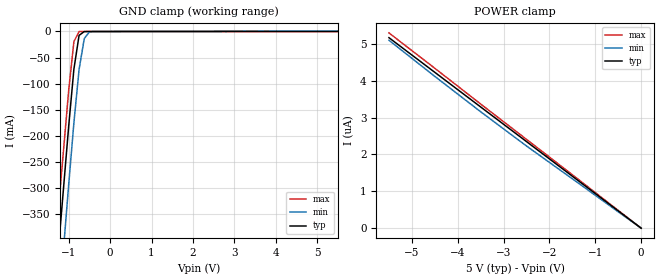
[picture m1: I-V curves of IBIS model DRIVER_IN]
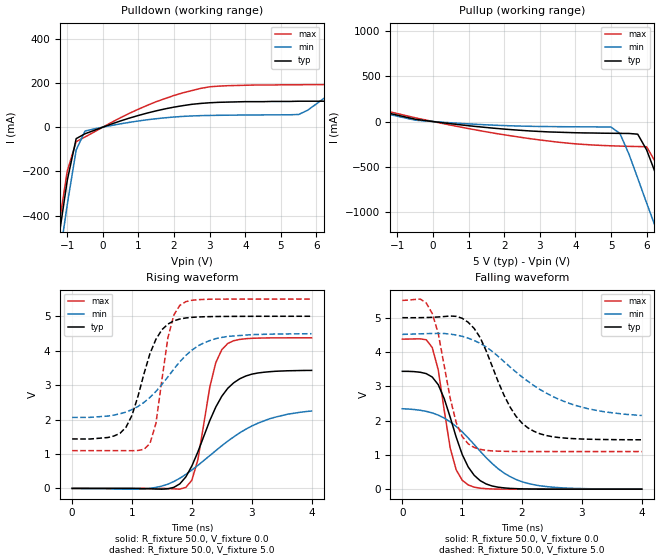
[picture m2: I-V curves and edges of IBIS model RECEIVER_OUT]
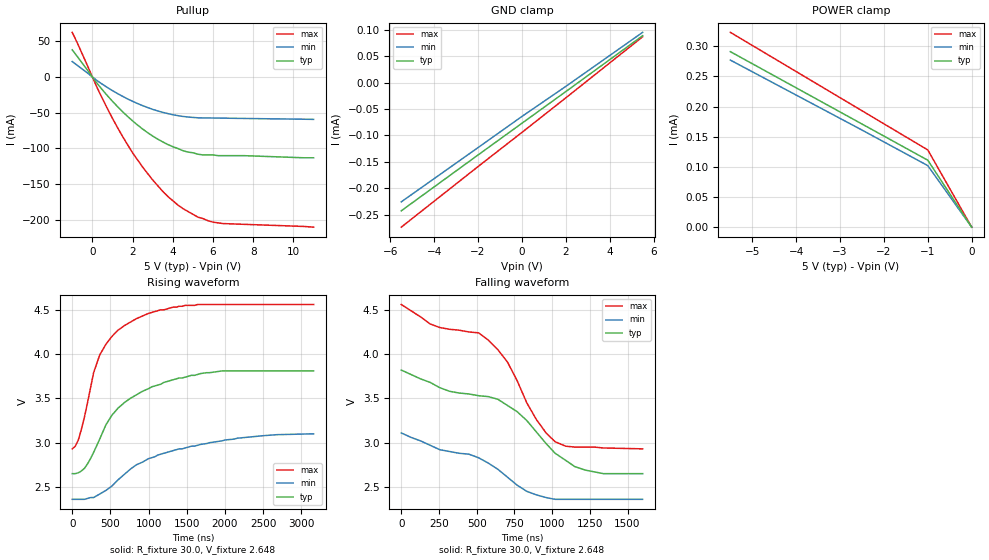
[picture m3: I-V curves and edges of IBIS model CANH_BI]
|   Texas Instruments Incorporated
|   Data Transmissions Products
|   IBIS Model for SN65HVD251
|   8D SOIC Package
[IBIS Ver]   3.2
[Comment char]   |_char
[File name]   hvd251100.ibs
[File Rev]   3.0
[Date]   23Oct02
[Source]   File originated at Texas Instruments Incorporated.
   Data Transmission Products Group.
[Notes]   RS is 100k
[Disclaimer]
(C) Copyright Texas Instruments Incorporated 2002
   All rights reserved
  Texas Instruments Incorporated hereby grants the user of this IBIS
model a non-exclusive, nontransferable license to use this IBIS model
under the following terms.  Before using this IBIS model, the user
should read this license.  If the user does not accept these terms,
the IBIS model should be returned to Texas Instruments within 30 days.
  The user is granted this license only to use the IBIS model and
is not granted rights to sell, load, rent, lease or license the IBIS
model in whole or in part, or in modified form to anyone other than
user.  User may modify the IBIS model to suit its specific applications
but rights to derivative works and such modifications shall belong to
Texas Instruments.
  This IBIS model is provided on an "AS IS" basis and Texas Instruments
makes absolutely no warranty with respect to the information contained
herein.  TEXAS INSTRUMENTS DISCLAIMS AND CUSTOMER WAIVES ALL WARRANTIES,
EXPRESS OR IMPLIED, INCLUDING WARRANTIES OF MERCHANTABILITY OR FITNESS
FOR A PARTICULAR PURPOSE. The entire risk as to quality and performance
is with the Customer. ACCORDINGLY, IN NO EVENT SHALL THE COMPANY BE LIABLE
FOR ANY DAMAGES, WHETHER IN CONTRACT OR TORT,INCLUDING ANY LOST PROFITS
OR OTHER INCIDENTAL, CONSEQUENTIAL, EXEMPLARY, OR PUNITIVE DAMAGES ARISING
OUT OF THE USE OR APPLICATION OF THE IBIS model provided in this package.
Further, Texas Instruments reserves the right to discontinue or make changes
without notice to any product herein to improve reliability, function, or
design. Texas Instruments does not convey any license under patent rights
or any other intellectual property rights, including those of third parties.
Contact Texas Instruments at ATTN:DATA TRANSMISSIONS
[Copyright]   Copyright 2002, Texas Instruments, All Rights Reserved
[Component]   HVD251D
[Manufacturer]  Texas Instruments Incorporated
[Package]
|   typ   min   max
R_pkg   0.036   0.033   0.039
L_pkg   3.340nH   2.445nH   4.233nH
C_pkg   0.470pF   0.308pF   0.631pF
[Pin]   signal_name   model_name   R_pin   L_pin   C_pin
1   D   DRIVER_IN   0.034   4.233n   0.630p
2   GND   GND   0.038   2.445n   0.309p
3   VCC   POWER   0.039   2.448n   0.309p
4   R   RECEIVER_OUT   0.033   4.231n   0.631p
5   NC   NC
6   CANL   CANL_BI   0.039   2.450n   0.308p
7   CANH   CANH_BI   0.039   2.448n   0.309p
8   NC   NC
[Diff_pin]   inv_pin   vdiff   tdelay_typ   tdelay_min   tdelay_max
| The CANL and CANH are Diff_pins
6   7   0.500   0 0 0
| Models and submodels in the file (4): DRIVER_IN (Input), RECEIVER_OUT (Output), CANH_BI (I/O_open_source), CANL_BI (I/O_open_drain)
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|   Driver Input Model
[Model]   DRIVER_IN
Model_type   Input
|Signals   D
Vinh = 2.0
Vinl = 0.8
|   typ   min   max
C_comp   1.0pF   NA   NA
|   typ   min   max
[Temperature Range]   25.0   -40   125
[Voltage Range]   5.0V   4.5V   5.5V
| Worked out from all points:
|   GND clamp passes 1 mA (typ) near -0.64 V on its own axis
[GND_clamp]
|   Voltage   I(typ)   I(min)   I(max)
-5.5V     -4.24A     -4.51A     -4.07A
-1.5V     -656mA     -786mA     -572mA
-1V       -181mA     -293mA     -112mA
-875mV    -72.1mA    -175mA     -19.3mA
-750mV    -7.44mA    -73mA      -168uA
-625mV    -113uA     -13.6mA    -58.6uA
-500mV    -28.2uA    -695uA     -58.3uA
5.5V      8.03uA     806uA      0A
[Power_clamp]
| Note that the[POWER_clamp]voltage table is referenced to Vcc
| and is calculated using Vtable=Vcc - Vmeasured.
|   Voltage   I(typ)   I(min)   I(max)
-5.5V     5.17uA     5.1uA      5.3uA
-4.5V     4.23uA     4.12uA     4.34uA
-3.5V     3.29uA     3.16uA     3.37uA
-2.5V     2.35uA     2.23uA     2.41uA
-1.5V     1.41uA     1.34uA     1.45uA
-500mV    469nA      444nA      482nA
0V        737fA      68.4pA     518fA
|   Receiver Output MODEL
[Model]   RECEIVER_OUT
Model_type   Output
| Signals   R
Vmeas = 2.4V   |Reference voltage for timing measurements
Cref = 15pF   |Timing specification test load capacitance value
| variable   typ   min   max
C_comp   1.0pF   NA   NA
|   typ   min   max
[Temperature Range]   25.0   -40   125
[Voltage Range]   5.0V   4.5V   5.5V
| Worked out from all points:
|   slope of the pulldown table from 0 to 0.75 V, typ, clamps not added: 18.3 ohm
|   slope of the pullup table from 0 to 0.75 V, typ, clamps not added: 21.1 ohm
|   rising waveform, R_fixture 50.0, V_fixture 0.0: 20-80 % time 520ps typ, 1.05ns min, 274ps max; typ from 0 V to 3.43 V
|   falling waveform, R_fixture 50.0, V_fixture 0.0: 20-80 % time 416ps typ, 835ps min, 254ps max; typ from 3.44 V to 0 V
|   rising waveform, R_fixture 50.0, V_fixture 5.0: 20-80 % time 384ps typ, 760ps min, 230ps max; typ from 1.44 V to 5 V
|   falling waveform, R_fixture 50.0, V_fixture 5.0: 20-80 % time 555ps typ, 1.13ns min, 308ps max; typ from 5 V to 1.44 V
[Pulldown]
|   Voltage   I(typ)   I(min)   I(max)
-5.5V     -5.08A     -5.12A     -5.12A
-1.5V     -784mA     -901mA     -716mA
-1V       -240mA     -349mA     -198mA
-750mV    -51.8mA    -103mA     -65.6mA
-500mV    -29.8mA    -17.4mA    -44.2mA
2.75V     107mA      51.9mA     175mA
5.5V      117mA      57.1mA     191mA
6.5V      125mA      166mA      193mA
7V        204mA      229mA      193mA
8V        381mA      356mA      357mA
9V        560mA      485mA      586mA
11V       921mA      742mA      1.05A
[Pullup]
|   Voltage   I(typ)   I(min)   I(max)
| Note that the[Pullup]voltage table is referenced to Vcc
| and is calculated using Vtable=Vcc - Vmeasured.
-5.5V     831mA      613mA      1.05A
-1.5V     116mA      103mA      135mA
-500mV    25.5mA     15.1mA     41.6mA
1.5V      -66.1mA    -36.3mA    -114mA
3.5V      -118mA     -56.7mA    -228mA
5V        -130mA     -60.7mA    -269mA
5.25V     -131mA     -133mA     -272mA
5.5V      -132mA     -358mA     -275mA
5.75V     -140mA     -628mA     -277mA
6V        -314mA     -903mA     -279mA
7.5V      -1.88A     -2.51A     -1.31A
11V       -5.61A     -6.16A     -5.12A
[Ramp]
|   typ   min   max
dV/dt_r   2.80V/700ps   1.87V/1400ps   3.51V/450ps
dV/dt_f   2.80V/750ps   1.88V/1550ps   3.51V/450ps
R_load = 50
[Rising Waveform]
R_fixture = 50.0
V_fixture = 0.0
C_fixture = 0p
L_fixture = 0n
|   V(typ)   V(min)   V(max)
0s        0V         0V         0V
1.6ns     -11mV      123mV      -4mV
1.9ns     335mV      409mV      30mV
2ns       652mV      534mV      238mV
2.1ns     1.058V     668mV      830mV
2.3ns     1.972V     954mV      2.947V
2.4ns     2.364V     1.098V     3.654V
2.5ns     2.677V     1.239V     4.029V
3ns       3.318V     1.811V     4.36V
4ns       3.428V     2.248V     4.374V
[Falling Waveform]
R_fixture = 50.0
V_fixture = 0.0
C_fixture = 0p
L_fixture = 0n
|   V(typ)   V(min)   V(max)
0s        3.436V     2.345V     4.374V
400ps     3.369V     2.269V     4.356V
500ps     3.269V     2.223V     4.13V
600ps     3.047V     2.159V     3.48V
800ps     2.097V     1.96V      1.198V
900ps     1.517V     1.828V     564mV
1.1ns     649mV      1.494V     125mV
1.4ns     152mV      920mV      14mV
2ns       9mV        216mV      0V
4ns       0V         2mV        0V
[Rising Waveform]
R_fixture = 50.0
V_fixture = 5.0
V_fixture_min = 4.5
V_fixture_max = 5.5
C_fixture = 0p
L_fixture = 0n
|   V(typ)   V(min)   V(max)
0s        1.437V     2.062V     1.097V
900ps     1.777V     2.216V     1.096V
1ns       2.123V     2.291V     1.095V
1.3ns     3.914V     2.643V     1.304V
1.4ns     4.333V     2.817V     1.89V
1.6ns     4.773V     3.239V     4.377V
1.7ns     4.868V     3.47V      5.04V
1.8ns     4.921V     3.681V     5.319V
2.4ns     4.993V     4.351V     5.497V
4ns       5V         4.494V     5.5V
[Falling Waveform]
R_fixture = 50.0
V_fixture = 5.0
V_fixture_min = 4.5
V_fixture_max = 5.5
C_fixture = 0p
L_fixture = 0n
|   V(typ)   V(min)   V(max)
0s        5V         4.513V     5.503V
300ps     5.001V     4.529V     5.543V
500ps     5.011V     4.54V      5.122V
900ps     5.039V     4.495V     1.943V
1.1ns     4.866V     4.404V     1.323V
1.3ns     4.42V      4.252V     1.161V
1.8ns     2.394V     3.563V     1.1V
2.1ns     1.785V     3.143V     1.097V
2.9ns     1.47V      2.439V     1.096V
4ns       1.44V      2.148V     1.097V
|   Driver (CANH) Output/Receiver Input Model
[Model]   CANH_BI
Model_type   I/O_open_source
| Signals   CANH
Vinh = 0.9V
Vinl = 0.5V
Rref = 30   |Note: 60 Ohm differential load;
Vref = 2.3   |tr and tf measured single-ended
| variable   typ   min   max
C_comp   1.0pF   NA   NA
|   typ   min   max
[Temperature Range]   25.0   -40   125
[Voltage Range]   5.0V   4.5V   5.5V
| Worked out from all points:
|   slope of the pullup table from 0 to 0.75 V, typ, clamps not added: 28.5 ohm
|   rising waveform, R_fixture 30.0, V_fixture 2.648: 20-80 % time 641ns typ, 1.01us min, 409ns max; typ from 2.65 V to 3.81 V
|   falling waveform, R_fixture 30.0, V_fixture 2.648: 20-80 % time 707ns typ, 572ns min, 381ns max; typ from 3.82 V to 2.65 V
[Pullup]
|   Voltage   I(typ)   I(min)   I(max)
| Note that the[Pullup]voltage table is referenced to Vcc
| and is calculated using Vtable=Vcc - Vmeasured.
-1V       37.9mA     21.5mA     62.4mA
500mV     -18mA      -10.2mA    -30.3mA
1.25V     -41.4mA    -23.2mA    -70.7mA
1.75V     -55.1mA    -30.7mA    -94.7mA
2.5V      -72.8mA    -40.1mA    -126mA
3V        -82.6mA    -45.3mA    -144mA
3.75V     -94.4mA    -51.2mA    -167mA
4.25V     -100mA     -54.1mA    -179mA
5.25V     -108mA     -57.1mA    -196mA
6V        -109mA     -57.4mA    -203mA
6.5V      -110mA     -57.6mA    -205mA
11V       -113mA     -59.3mA    -210mA
[Power_clamp]
| Note that the[POWER_clamp]voltage table is referenced to Vcc
| and is calculated using Vtable=Vcc - Vmeasured.
|   Voltage   I(typ)   I(min)   I(max)
-5.5V     291uA      277uA      323uA
-4V       231uA      219uA      258uA
-2.5V     171uA      161uA      193uA
-1V       111uA      102uA      128uA
0V        0A         0A         0A
[GND_clamp]
|   Voltage   I(typ)   I(min)   I(max)
-5.5V     -243uA     -226uA     -274uA
-2V       -137uA     -123uA     -159uA
0V        -76.8uA    -63.9uA    -94.2uA
2V        -16.7uA    -6.87uA    -28.6uA
5.5V      89.3uA     95.7uA     87.3uA
[Ramp]
|   typ   min   max
dV/dt_r   1.17/1080ns   0.75/1600ns   1.63/720ns
dV/dt_f   1.17/960ns   0.75/736ns   1.63/800ns
R_load = 30ohm  | Note: The measurement is single-ended with 30ohm
|   to V_fixture
[Rising Waveform]
R_fixture = 30.0
V_fixture = 2.648
V_fixture_min = 2.356
V_fixture_max = 2.927
C_fixture = 0p
L_fixture = 0n
|   V(typ)   V(min)   V(max)
0s        2.65V      2.36V      2.93V
80ns      2.66V      2.36V      3.03V
160ns     2.71V      2.36V      3.29V
280ns     2.89V      2.38V      3.79V
360ns     3.04V      2.42V      3.99V
520ns     3.31V      2.51V      4.2V
680ns     3.45V      2.64V      4.32V
1us       3.61V      2.82V      4.46V
1.68us    3.78V      2.98V      4.56V
3.16us    3.81V      3.1V       4.56V
[Falling Waveform]
R_fixture = 30.0
V_fixture = 2.648
V_fixture_min = 2.356
V_fixture_max = 2.927
C_fixture = 0p
L_fixture = 0n
|   V(typ)   V(min)   V(max)
0s        3.82V      3.11V      4.56V
192ns     3.68V      2.97V      4.34V
512ns     3.53V      2.83V      4.24V
576ns     3.52V      2.77V      4.16V
704ns     3.42V      2.61V      3.91V
768ns     3.35V      2.52V      3.7V
896ns     3.12V      2.41V      3.26V
1.02us    2.88V      2.36V      3.01V
1.22us    2.69V      2.36V      2.95V
1.6us     2.65V      2.36V      2.93V
